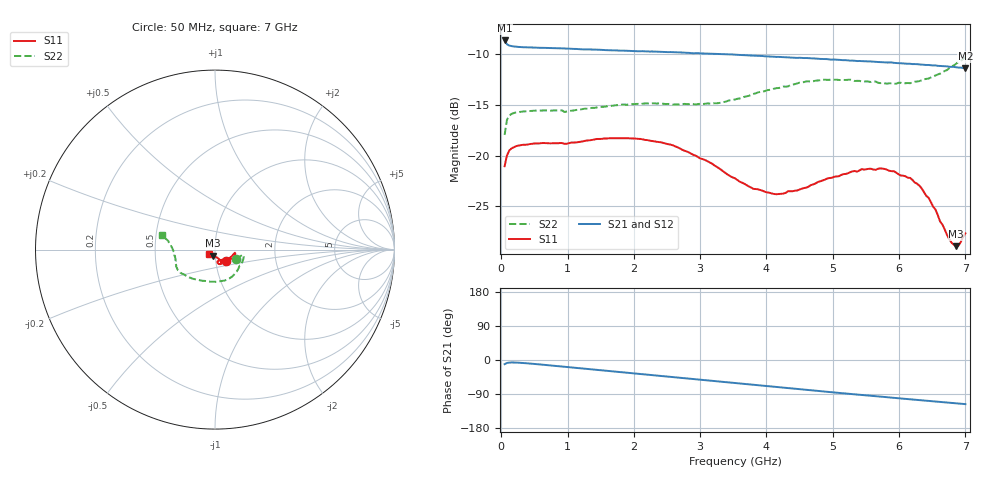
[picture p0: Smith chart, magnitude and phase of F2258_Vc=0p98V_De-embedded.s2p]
! Integrated Device Technology
! Corporate Headquarters
! 6024 Silver Creek Valley Road
! San Jose, CA 95138  USA
! Phone:  1-408-284-8200
! Toll Free:  1-800-223-1366
! Webpage:  http://www.idt.com/
! Timing and RF Division
! 515 Groton Road, Suite 102
! Westford, MA 01886-6024
! Device:  F2258
! Description: Voltage Variable RF Attenuator
! Frequency:  50.0 -  6000.00 MHz
! Package:  3x3 mm Thin QFN Plastic Package: 16 pin
! Ports:  2 RF, 2 DC
!  Pin  1  = NC
!  Pin  2  = NC
!  Pin  3  = RF2  = Port 2
!  Pin  4  = GND
!  Pin  5  = Vdd
!  Pin  6  = NC
!  Pin  7  = VCTRL
!  Pin  8  = NC
!  Pin  9  = GND
!  Pin 10  = RF1  = Port 1
!  Pin 11  = NC
!  Pin 12  = NC
!  Pin 13  = NC
!  Pin 14  = NC
!  Pin 15  = NC
!  Pin 16  = NC
! Vcntrl:  0.980 Volts
! Vdd:  +3.300 Volts
! Current:  1.155 mA
! Data:  The device was measured on a the F2258 evaluation board which has
!  individual transmission lines to the RF pins.  Data was collected
!  using a calibrated network analyzer.  The evaluation board was
!  de-embedded using a TRL calibration technique.
!  The reference plane is the edge of the package pin.
! Misc:  SN 10
!  Action Tracker AT0285
! Date Measured:  2014-12-10
! Date:  2016-01-13  MJV
! Note:
!  Integrated Device Technology supplies this data as a sample of measured
!  data at the package pin for this product.  Your particular data for this
!  product may vary.
!  Data was taken at 25 degrees C.
!  Integrated Device Technology reserves the right to change this data at anytime.
!Freq_(GHz)  S11M_(dB)  S11P_(deg)  S21M_(dB)  S21P_(deg)  S12M_(dB)  S12P_(deg)  S22M_(dB)  S22P_(deg)
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# GHz S dB R 50
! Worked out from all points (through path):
!   201 points, 50 MHz to 7 GHz, reference 50 ohm
!   highest |S21| = -8.66 dB at 50 MHz (marker M1); lowest = -11.4 dB at 7 GHz (marker M2)
!   group delay of S21, straight-line fit = 45.6 ps
!   lowest |S11| = -28.9 dB at 6.861 GHz (marker M3), VSWR 1.07, Z = 48.6 - j3.24 ohm
!   |S11| at or under -10 dB: start of sweep to end of sweep
!   |S22| runs from -18.0 to -10.3 dB; largest |S21 - S12| = 0.0014
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0.05  -21.05 -45.2  -8.66 -11.0  -8.64 -10.9  -17.97 -24.1
0.08475  -20.01 -22.3  -9.03 -7.9  -9.02 -7.9  -16.51 -13.2
0.1195  -19.51 -15.0  -9.16 -6.8  -9.15 -6.8  -16.07 -11.0
0.189  -19.18 -10.6  -9.25 -6.5  -9.25 -6.5  -15.81 -10.6
1.2315  -18.61 -19.7  -9.54 -22.5  -9.53 -22.5  -15.41 -41.4
1.82225  -18.28 -23.5  -9.66 -32.3  -9.65 -32.3  -14.98 -57.4
2.37825  -18.68 -25.9  -9.78 -41.5  -9.78 -41.5  -14.86 -72.7
2.58675  -18.99 -27.8  -9.81 -45.0  -9.82 -45.0  -14.99 -78.8
3.07325  -20.44 -33.5  -9.94 -53.3  -9.92 -53.3  -14.90 -96.5
3.525  -22.25 -44.9  -10.06 -61.0  -10.04 -61.0  -14.48 -114.7
3.803  -23.29 -56.3  -10.16 -65.7  -10.13 -65.8  -13.93 -125.2
4.1505  -23.82 -68.3  -10.28 -71.5  -10.24 -71.6  -13.36 -135.6
4.7065  -22.85 -78.7  -10.43 -80.7  -10.44 -80.7  -12.68 -148.2
5.43625  -21.34 -72.0  -10.69 -92.2  -10.69 -92.2  -12.70 -159.7
5.85325  -21.51 -65.2  -10.83 -98.8  -10.83 -98.8  -12.88 -168.2
6.166  -22.21 -62.9  -10.96 -103.7  -10.96 -103.7  -12.87 -175.5
6.33975  -23.23 -62.8  -11.03 -106.5  -11.03 -106.5  -12.59 179.6
6.54825  -25.33 -69.1  -11.12 -109.8  -11.13 -109.7  -12.11 174.4
6.75675  -28.23 -90.3  -11.25 -113.0  -11.26 -112.9  -11.39 169.0
6.861  -28.94 -111.2  -11.30 -114.5  -11.31 -114.4  -10.95 167.2
6.89575  -28.89 -120.1  -11.33 -114.9  -11.34 -115.0  -10.77 166.5
7  -27.68 -142.5  -11.38 -116.5  -11.40 -116.5  -10.29 164.5
